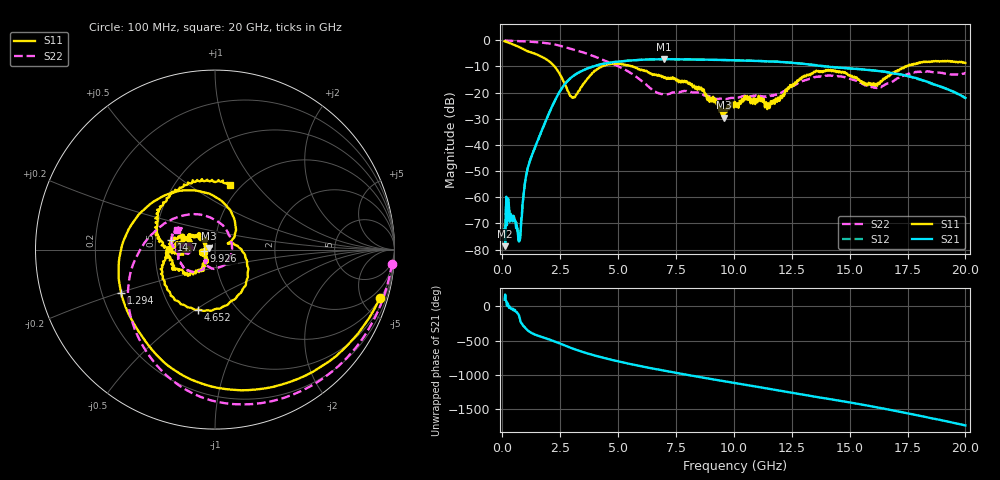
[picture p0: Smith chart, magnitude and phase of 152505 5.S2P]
!  2-Port S-parameters saved by WinCal
! VAR MeasName=S-Parameters (CALIBRATED_DATA) read from VNA (N5230C)
! VAR MeasDate=4/10/2015 9:28:54 AM
! VAR NAME=152505 5
! VAR FILENAME=152505 5.S2P
! VAR DATE=4/10/2015 9:28:55 AM
! VAR PHYS_PORTS=1,2
# Hz S DB R 50
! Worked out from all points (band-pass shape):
!   801 points, 100 MHz to 20 GHz, reference 50 ohm
!   highest |S21| = -7.22 dB at 6.99 GHz (marker M1); lowest = -78.7 dB at 124.9 MHz (marker M2)
!   |S21| within 3 dB of the highest: 3.853 GHz to 14.19 GHz (10.33 GHz wide, 115 % of centre)
!   lowest |S11| = -29.6 dB at 9.577 GHz (marker M3), VSWR 1.07, Z = 46.9 + j0.732 ohm
!   |S11| at or under -10 dB: 2.253 GHz to 4.302 GHz (2.049 GHz wide, 62.5 % of centre); 5.632 GHz to 17.46 GHz (11.83 GHz wide, 102 % of centre)
!   |S22| runs from -22.5 to -0.1 dB; largest |S21 - S12| = 0.0069
!   S11 on the Smith chart (normalised r, x): 100 MHz: 1.04, -6.81; 1.294 GHz: 0.28, -0.20; 4.652 GHz: 0.67, -0.51; 9.926 GHz: 0.88, -0.02; 14.7 GHz: 0.61, +0.07; 20 GHz: 0.89, +0.74
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1e8  -0.37 -16.3  -72.18 96.8  -70.06 121.8  -0.08 -4.6
1.24875e8  -0.46 -20.0  -78.70 171.2  -73.26 137.0  -0.11 -5.5
2.74125e8  -0.92 -41.0  -61.96 -7.0  -62.79 -7.5  -0.17 -11.5
7.4675e8  -2.66 -100.3  -76.65 -164.9  -73.56 -157.0  -0.35 -30.3
1.020375e9  -3.95 -129.1  -52.15 36.3  -52.15 35.4  -0.46 -41.3
1.294e9  -4.79 -155.3  -43.66 -33.2  -43.69 -33.2  -0.60 -52.4
2.065125e9  -8.34 121.2  -26.95 -127.7  -26.97 -127.7  -1.31 -85.3
3.010375e9  -21.88 26.2  -14.02 108.5  -14.02 108.6  -3.38 -125.3
3.43325e9  -17.71 7.2  -11.75 59.3  -11.73 59.6  -4.49 -142.3
4.652125e9  -9.19 -105.4  -8.59 -54.0  -8.55 -53.9  -8.61 168.9
5.497875e9  -9.65 -155.8  -7.78 -118.1  -7.73 -118.3  -12.24 126.8
6.741625e9  -13.21 170.1  -7.26 157.8  -7.23 157.4  -20.26 13.4
6.990375e9  -14.40 169.4  -7.22 141.8  -7.27 141.7  -20.64 -17.8
8.134625e9  -17.04 147.5  -7.33 72.7  -7.36 72.7  -19.80 -107.5
9.577375e9  -29.60 166.4  -7.57 -10.7  -7.58 -10.4  -22.31 -131.0
9.925625e9  -24.11 -171.7  -7.61 -30.4  -7.61 -30.4  -22.02 -125.8
1.005e10  -23.56 -162.8  -7.63 -37.6  -7.65 -37.7  -21.98 -126.8
1.204e10  -21.24 -120.8  -8.31 -151.0  -8.32 -151.1  -20.04 -122.1
1.338325e10  -12.68 -149.6  -9.43 131.3  -9.37 131.5  -14.36 -141.9
1.470162e10  -12.08 167.2  -10.57 57.8  -10.55 56.6  -13.95 179.4
1.669162e10  -13.66 -171.4  -12.31 -63.9  -12.32 -64.9  -16.44 -171.0
2e10  -8.68 76.8  -22.05 65.2  -22.09 65.8  -12.54 153.2
